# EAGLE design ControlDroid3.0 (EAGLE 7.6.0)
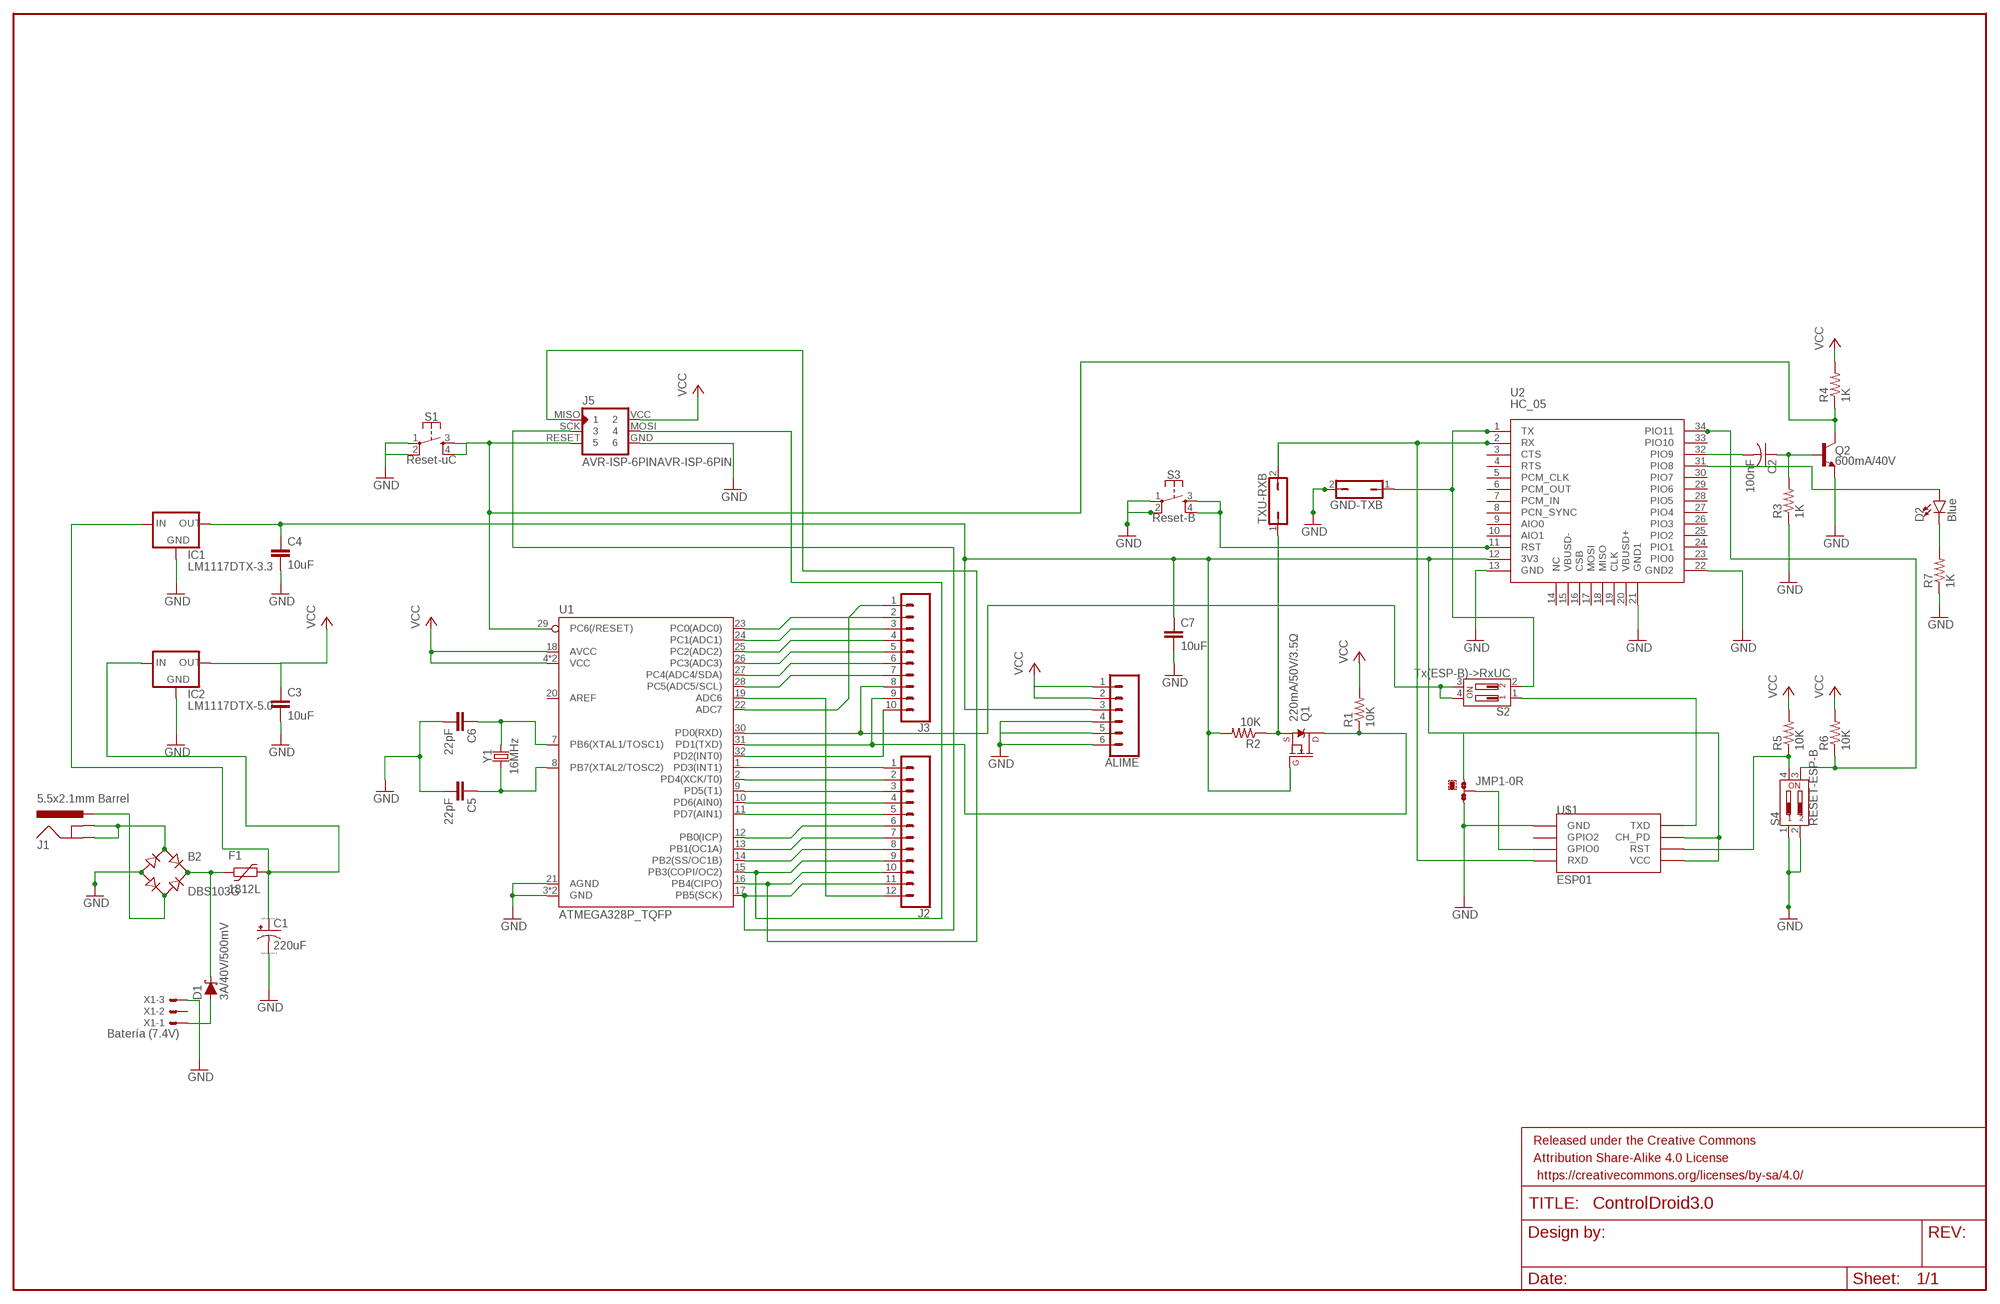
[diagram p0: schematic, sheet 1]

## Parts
ALIME  CONN_06NO_SILK_FEMALE_PTH  [1X06_NO_SILK]
B2  DBS103G  [DBS]
C1  220uF  CPOL-US153CLV-0605  [153CLV-0605]
C2  100nF  C-USC0805  [C0805]
C3  10uF  10UF-1206-6.3V-20%  [1206]
C4  10uF  10UF-1206-6.3V-20%  [1206]
C5  22pF  22PF-0603-50V-5%  [0603]
C6  22pF  22PF-0603-50V-5%  [0603]
C7  10uF  10UF-1206-6.3V-20%  [1206]
D1  3A/40V/500mV  DIODE-SCHOTTKY-B340A  [SMA-DIODE]
D2  Blue  LED-BLUE1206  [LED-1206]
F1  1812L  [1812L]
FRAME1  FRAME-LEDGERNO_FOOTPRINT  [DUMMY]
GND-TXB  JP1Q  [JP1]
IC1  LM1117DTX-3.3  [TO252]
IC2  LM1117DTX-5.0  [TO252]
J1  5.5x2.1mm Barrel  POWER_JACKSMD  [POWER_JACK_SMD]
J2  CONN_12  [1X12]
J3  CONN_10"  [1X10]
J5  AVR-ISP-6PINAVR-ISP-6PIN  [AVR-ISP-6PIN]
JMP1  0R-JUMPA  [A0R-JMP]
Q1  220mA/50V/3.5Ω  MOSFET-NCH-BSS138  [SOT23-3]
Q2  600mA/40V  TRANS_NPN-MMBT2222AL  [SOT23-3]
R1  10K  R-US_R1206  [R1206]
R2  10K  R-US_R1206  [R1206]
R3  1K  R-US_R1206  [R1206]
R4  1K  R-US_R1206  [R1206]
R5  10K  R-US_R1206  [R1206]
R6  10K  R-US_R1206  [R1206]
R7  1K  R-US_R1206  [R1206]
S1  Reset-uC  MOMENTARY-SWITCH-SPST-2-SMD-5.2MM  [TACTILE_SWITCH_SMD_5.2MM]
S2  Tx(ESP-B)->RxUC  DIP-02-SMD-50MIL-JWING  [DIPSWITCH-02-CHS-02A]
S3  Reset-B  MOMENTARY-SWITCH-SPST-2-SMD-5.2MM  [TACTILE_SWITCH_SMD_5.2MM]
S4  RESET-ESP-B  DIP-02-SMD-50MIL-JWING  [DIPSWITCH-02-CHS-02A]
TXU-RXB  JP1Q  [JP1]
U1  ATMEGA328P_TQFP  [TQFP32-08]
U2  HC_05  [BLUETOOTH_SMD]
U$1  ESP01  [ESP01]
X1  Batería (7.4V)  C-GRID-03-70543  [70543-03]
Y1  16MHz  CRYSTAL-8MHZSMD-HC49UP  [HC49UP]

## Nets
GND: ALIME.4 ALIME.5 ALIME.6 B2.- C1.- C3.2 C4.2 C5.2 C6.2 C7.2 GND-TXB.2 IC1.1(GND) IC2.1(GND) J5.GND JMP1.3 Q2.2(E) R3.1 R7.1 S1.1 S1.2 S3.1 S3.2 S4.1 S4.2 U1.3(GND) U1.5(GND) U1.21(AGND) U2.13(GND) U2.21(GND1) U2.22(GND2) U$1.GND X1.3
N$1: C6.1 U1.7(PB6(XTAL1/TOSC1)) Y1.2
N$2: B2.AC2 J1.VIN0(PWR)
N$3: B2.AC1 J1.GND(GNDBREAK) J1.P$4(GND)
N$4: B2.+ D1.C F1.P$1
N$6: C1.+ F1.P$2 IC1.2(IN) IC2.2(IN)
N$7: C5.1 U1.8(PB7(XTAL2/TOSC2)) Y1.1
N$8: J2.1 U1.1(PD3(INT1))
N$9: J2.2 U1.2(PD4(XCK/T0))
N$10: J2.3 U1.9(PD5(T1))
N$11: J2.4 U1.10(PD6(AIN0))
N$12: J2.5 U1.11(PD7(AIN1))
N$13: J2.6 U1.12(PB0(ICP))
N$14: J2.7 U1.13(PB1(OC1A))
N$15: J2.8 U1.14(PB2(SS/OC1B))
N$16: J2.9 J5.MOSI U1.15(PB3(COPI/OC2))
N$17: J3.9 Q1.3(D) R1.1 U1.31(PD1(TXD))
N$18: J2.11 J5.SCK U1.17(PB5(SCK))
N$19: J2.12 U1.19(ADC6)
N$20: J3.1 U1.22(ADC7)
N$21: J3.2 U1.23(PC0(ADC0))
N$22: J3.3 U1.24(PC1(ADC1))
N$23: J3.4 U1.25(PC2(ADC2))
N$24: J3.5 U1.26(PC3(ADC3))
N$25: J3.6 U1.27(PC4(ADC4/SDA))
N$26: J3.7 U1.28(PC5(ADC5/SCL))
N$27: S2.1 U$1.TX(TXD)
N$28: J3.8 S2.3 S2.4 U1.30(PD0(RXD))
N$29: J3.10 U1.32(PD2(INT0))
N$30: Q1.2(S) R2.1 TXU-RXB.1
N$32: J5.RESET Q2.3(C) R4.1 S1.3 S1.4 U1.29(PC6(/RESET))
N$35: D1.A X1.1
N$36: ALIME.3 C4.1 C7.1 IC1.TAB(OUT) JMP1.1 Q1.1(G) R2.2 U2.12(3V3) U$1.CH_PD U$1.VCC
N$37: J2.10 J5.MISO U1.16(PB4(CIPO))
N$38: GND-TXB.1 S2.2 U2.1(TX)
N$39: TXU-RXB.2 U2.2(RX) U$1.RX(RXD)
N$40: S3.3 S3.4 U2.11(RST)
N$41: C2.2 U2.32(PIO9)
N$42: C2.1 Q2.1(B) R3.2
N$43: R5.1 S4.4 U$1.RST
N$44: R6.1 S4.3 U2.34(PIO11)
N$45: D2.A U2.31(PIO8)
N$46: D2.C R7.2
N$47: JMP1.2 U$1.GPIO0
VCC: ALIME.1 ALIME.2 C3.1 IC2.TAB(OUT) J5.VCC R1.2 R4.2 R5.2 R6.2 U1.4(VCC) U1.6(VCC) U1.18(AVCC)
Unconnected: U1.20(AREF) U2.3(CTS) U2.4(RTS) U2.5(PCM_CLK) U2.6(PCM_OUT) U2.7(PCM_IN) U2.8(PCN_SYNC) U2.9(AIO0) U2.10(AIO1) U2.14(NC) U2.15(VBUSD-) U2.16(CSB) U2.17(MOSI) U2.18(MISO) U2.19(CLK) U2.20(VBUSD+) U2.23(PIO0) U2.24(PIO1) U2.25(PIO2) U2.26(PIO3) U2.27(PIO4) U2.28(PIO5) U2.29(PIO6) U2.30(PIO7) U2.33(PIO10) U$1.GPIO2 X1.2

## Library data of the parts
ALIME = SparkFun-Connectors:CONN_06: Multi connection point. Often used as Generic Header-pin footprint for 0.1 inch spaced/style header connections On any of the 0.1 inch spaced packages, you can populate with these: Break Away Headers - Straight (PRT-00116) Break Away Male Headers - Right Angle (PRT-00553) Female Headers (PRT-00115)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; PROD_ID: CONN-08437
B2 = rectifier:DB?*G: Single Phase 1.0 AMP Glass Passivated Bridge Rectifier Taiwan Semiconductor Co.,Ltd. - TSC Source: http://www.taiwansemi.com/TSCbig5/ezcatfiles/cust/img/img/db101g.pdf http://www.ts.com.tw/db/pictures/modules/PDT/PDT060207001/DBLS201G.pdf
C1 = resistor:CPOL-US: POLARIZED CAPACITOR, American symbol
C2 = rcl:C-US: CAPACITOR, American symbol
C3 C4 C7 = SparkFun-Capacitors:10UF: 10.0µF ceramic capacitors; PROD_ID: CAP-10057
C5 C6 = SparkFun-Capacitors:22PF: 22pF ceramic capacitors; PROD_ID: CAP-07876
D1 = SparkFun-DiscreteSemi:DIODE-SCHOTTKY: Schottky diode; PROD_ID: DIO-09886
D2 = SparkFun-LED:LED-BLUE: Blue SMD LED; PROD_ID: DIO-09911
F1 = ptc-littlefuse:1812L
FRAME1 = SparkFun-Aesthetics:FRAME-LEDGER: Schematic Frame - Ledger
GND-TXB TXU-RXB = jumper:JP1Q: JUMPER
IC1 IC2 = lm1117:LM1117DTX-*
J1 = SparkFun-Connectors:POWER_JACK: Power Jack Connector This is the standard 5.5mm barrel jack for power. The PTH is the most common, proven, reliable, footprint. The Slot footprint only works if the mill layer is transmitted to the PCB fab house so be warned. Here are the connectors we sell at SparkFun: DC Barrel Power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; PROD_ID: CONN-08106; SF_ID: PRT-12748
J2 = SparkFun-Connectors:CONN_12: Multi connection point. Often used as Generic Header-pin footprint for 0.1 inch spaced/style header connections On any of the 0.1 inch spaced packages, you can populate with these: Break Away Headers - Straight (PRT-00116) Break Away Male Headers - Right Angle (PRT-00553) Female Headers (PRT-00115)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
J3 = SparkFun-Connectors:CONN_10: Multi connection point. Often used as Generic Header-pin footprint for 0.1 inch spaced/style header connections On any of the 0.1 inch spaced packages, you can populate with these: Break Away Headers - Straight (PRT-00116) Break Away Male Headers - Right Angle (PRT-00553) Female Headers (PRT-00115)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; PROD_ID: CONN-11563
J5 = avr-isp:AVR-ISP-6PIN: AVR ISP 6pin 3x2 pin header
JMP1 = jump-0r-smd:0R-JUMP: SMD 0R 0805 Jumper
Q1 = SparkFun-DiscreteSemi:MOSFET-NCH: N-channel MOSFETs Voltage controlled devices that allow control of high current outputs. SparkFun Products: SparkFun OpenScale SparkFun Digital Sandbox SparkFun Monster Moto Shield SparkFun MOSFET Power Controller; PROD_ID: TRANS-00830
Q2 = SparkFun-DiscreteSemi:TRANS_NPN: NPN transistor Current controlled devices typically used to amplify current or used as a switch. BC547 - COM-08928 (TO-92 45V 100mA) (1.Collector 2.Base 3.Emitter) 2N3904 - COM-00521 (TO-92 40V 200mA) (1.Emitter 2.Base 3.Collector) P2N2222A - COM-12852 (TO-92 40V 600mA) (1.Collector 2.Base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; PROD_ID: TRANS-08049
R1-R7 = resistor:R-US_: RESISTOR, American symbol
S1 S3 = SparkFun-Switches:MOMENTARY-SWITCH-SPST-2: Momentary Switch (Pushbutton) - SPST - Two Circuits Normally-open (NO) SPST momentary switches (buttons, pushbuttons). Schematic symbol includes two switch circuits. Variants SMD-4.6MMX2.8MM - 4.60mm x 2.80mm Tactile Momentary Button Switch - Used on SparkFun Pro Micro - RP2040 SMD-5.2MM - Mini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; PROD_ID: SWCH-08247; SF_SKU: COM-08720
S2 S4 = SparkFun-Switches:DIP-02: 2-Position DIP Switch 2-circuit DIP (dual inline package) switch. Commonly used to physcially set a circuit's behavior. Variants PTH-100MIL - Through-hole, 0.1"-Pitch Used on SparkFun Stepoko (ROB-13899) SMD-50MIL-JWING - SMD (J-Wing Pads), 0.05"-Pitch Prototype Part SMD-50MIL - SMD, 0.05"-Pitch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; PROD_ID: SWCH-12372
U1 = SparkFun-IC-Microcontroller:ATMEGA328P_TQFP: Popular 328P in QFP Storefront component: ATmega328 - TQFP (COM-13448) Datasheet SparkFun Products SparkFun RedBoard - Programmed with Arduino (DEV-12757) Arduino Pro Mini 328 - 5V/16MHz (DEV-11113) Arduino Pro Mini 328 - 3.3V/8MHz (DEV-11114) SparkFun OpenLog (DEV-13712) SparkFun MicroView - OLED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; PROD_ID: IC-09069
U2 = Bluetooth HC-05:HC_05: HC-05 Bluetooth Module
U$1 = esp8266modules:ESP01: ESP8266 Wifi module 01
X1 = con-molex:C-GRID-03: CONNECTOR wire to board 2.54 mm (0.100") pitch header; OC_FARNELL: unknown; OC_NEWARK: unknown
Y1 = SparkFun-Clocks:CRYSTAL-8MHZ: 8MHz Crystal; PROD_ID: XTAL-11706; VALUE: 8MHz

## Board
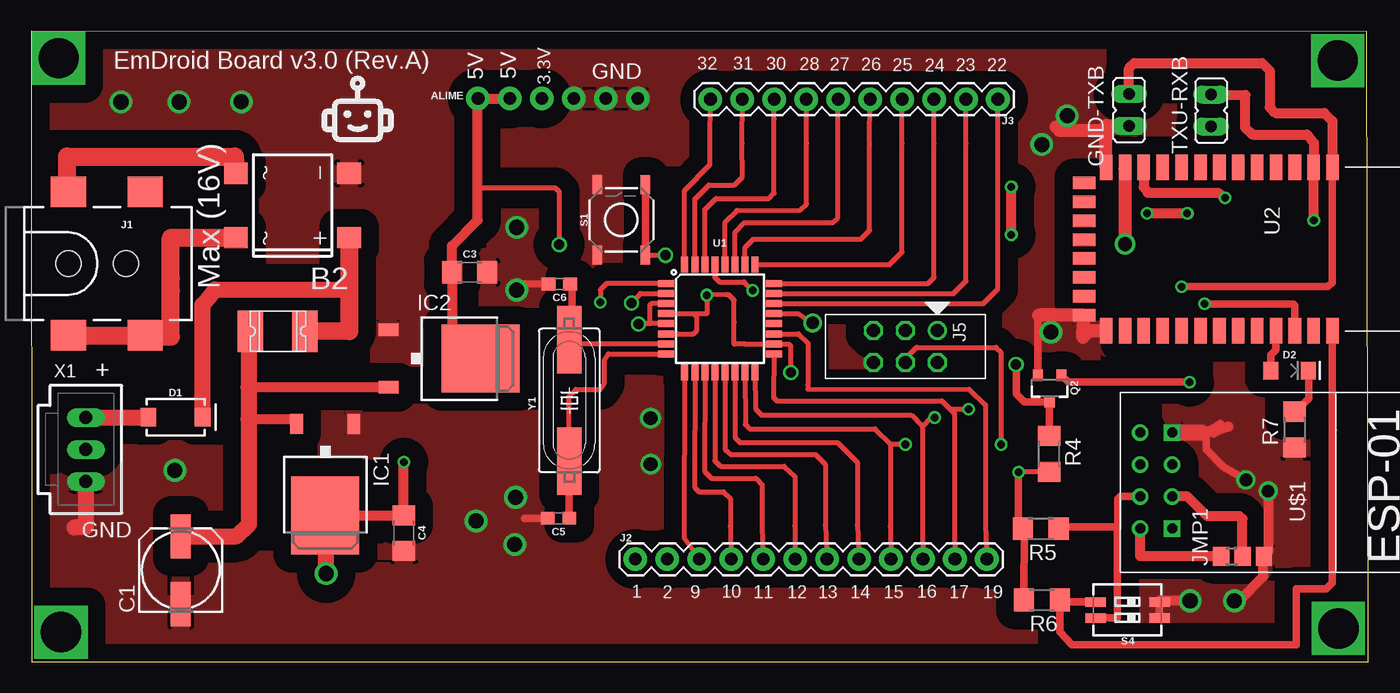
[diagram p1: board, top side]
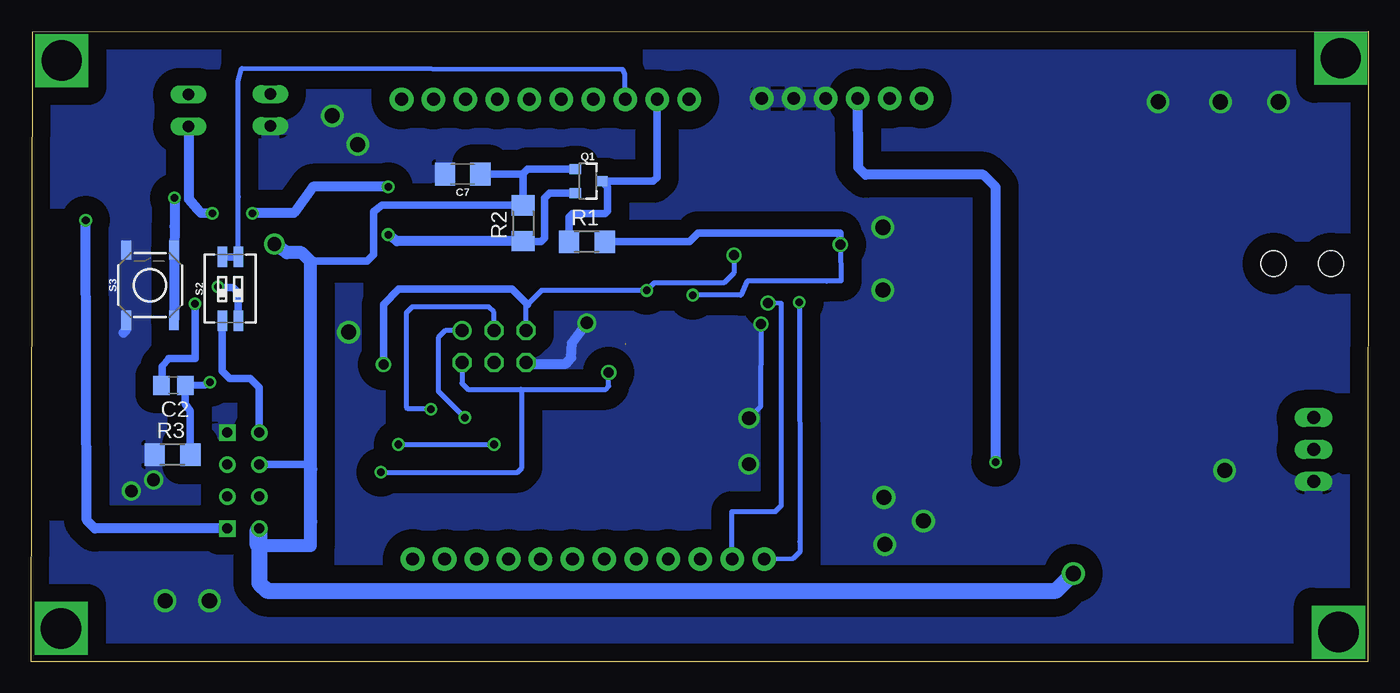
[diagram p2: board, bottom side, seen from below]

Size 106.24 x 50.1 mm. Coordinates in mm from the lower left corner, seen from the top.
Outline: 0,0 106.24,0 106.15,50.06 0,50.1 0,0
Copper layers (1*16): Top 0.035mm / dielectric 1.5mm / Bottom 0.035mm
Design rules "default *": minimum track width 10mil, minimum drill 16mil, track to track 8mil, track to pad 8mil, pad to pad 8mil, via to via 8mil, smd to smd 8mil, copper to edge 40mil, drill to drill 8mil, minimum pad ring 10mil, minimum via ring 8mil, stop-mask expansion 4mil, vias tented up to drill 0mil, thermal gap 10mil

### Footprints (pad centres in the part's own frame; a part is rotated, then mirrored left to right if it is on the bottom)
1X06_NO_SILK = drill 1.016 pad 1.88: 1 0,0; 2 2.54,0; 3 5.08,0; 4 7.62,0; 5 10.16,0; 6 12.7,0
DBS = smd 1.7 x 1.9: + -2.55,-4.5; - 2.55,-4.5; AC1 -2.55,4.5; AC2 2.55,4.5
153CLV-0605 = smd 3.5 x 1.6: + 2.7,0; - -2.7,0
C0805 = smd 1.3 x 1.5: 1 -0.95,0; 2 0.95,0
1206 = smd 1.6 x 1.8: 1 -1.4,0; 2 1.4,0
0603 = smd 1.1 x 1: 1 -0.85,0; 2 0.85,0
SMA-DIODE = smd 1.27 x 1.47: A -2.15,0; C 2.15,0
LED-1206 = smd 1.2 x 1.4: A -1.5,0; C 1.5,0
1812L = smd 2.03 x 3.3: P$1 -2.16,0; P$2 2.16,0
JP1 = drill 0.914 long: 1 0,-1.27; 2 0,1.27
TO252 = smd 1 x 1.6: 1 -2.28,-4.8; 2 2.28,-4.8 | smd 5.4 x 6.2: TAB 0,2.5
POWER_JACK_SMD = smd 2.8 x 2.4: GND 0,-5.7; P$4 6.1,-5.7; VIN0 0,5.7; VIN1 6.1,5.7 | hole 2.032: 0,0; 4.572,0
1X12 = drill 1.016 pad 1.88: 1 0,0; 2 2.54,0; 3 5.08,0; 4 7.62,0; 5 10.16,0; 6 12.7,0; 7 15.24,0; 8 17.78,0; 9 20.32,0; 10 22.86,0; 11 25.4,0; 12 27.94,0
1X10 = drill 1.016 pad 1.88: 1 0,0; 2 2.54,0; 3 5.08,0; 4 7.62,0; 5 10.16,0; 6 12.7,0; 7 15.24,0; 8 17.78,0; 9 20.32,0; 10 22.86,0
AVR-ISP-6PIN = drill 1.016 octagon: GND 1.27,-2.54; MOSI 1.27,0; RESET -1.27,-2.54; SCK -1.27,0; VCC 1.27,2.54 | drill 1.016: MISO -1.27,2.54
A0R-JMP = smd 1.5 x 1.3: 1 0,1.7; 2 0,0; 3 0,-1.7
SOT23-3 = smd 0.8 x 0.9: 1 -0.95,-1; 2 0.95,-1; 3 0,1.1
R1206 = smd 1.6 x 1.803: 1 -1.422,0; 2 1.422,0
TACTILE_SWITCH_SMD_5.2MM = smd 1.524 x 0.762: 1 -2.794,1.905; 2 2.794,1.905; 3 -2.794,-1.905; 4 2.794,-1.905
DIPSWITCH-02-CHS-02A = smd 0.76 x 1.6: 1 0,-2.54; 2 1.27,-2.54; 3 1.27,2.54; 4 0,2.54
TQFP32-08 = smd 1.27 x 0.559: 1 -4.293,2.8; 2 -4.293,2; 3 -4.293,1.2; 4 -4.293,0.4; 5 -4.293,-0.4; 6 -4.293,-1.2; 7 -4.293,-2; 8 -4.293,-2.8; 17 4.293,-2.8; 18 4.293,-2; 19 4.293,-1.2; 20 4.293,-0.4; 21 4.293,0.4; 22 4.293,1.2; 23 4.293,2; 24 4.293,2.8 | smd 0.559 x 1.27: 9 -2.8,-4.293; 10 -2,-4.293; 11 -1.2,-4.293; 12 -0.4,-4.293; 13 0.4,-4.293; 14 1.2,-4.293; 15 2,-4.293; 16 2.8,-4.293; 25 2.8,4.293; 26 2,4.293; 27 1.2,4.293; 28 0.4,4.293; 29 -0.4,4.293; 30 -1.2,4.293; 31 -2,4.293; 32 -2.8,4.293
BLUETOOTH_SMD = smd 2 x 1: 1 -6.35,3.81; 2 -6.35,2.31; 3 -6.35,0.81; 4 -6.35,-0.69; 5 -6.35,-2.19; 6 -6.35,-3.69; 7 -6.35,-5.19; 8 -6.35,-6.69; 9 -6.35,-8.19; 10 -6.35,-9.69; 11 -6.35,-11.19; 12 -6.35,-12.69; 13 -6.35,-14.19; 22 6.65,-14.19; 23 6.65,-12.69; 24 6.65,-11.19; 25 6.65,-9.69; 26 6.65,-8.19; 27 6.65,-6.69; 28 6.65,-5.19; 29 6.65,-3.69; 30 6.65,-2.19; 31 6.65,-0.69; 32 6.65,0.81; 33 6.65,2.31; 34 6.65,3.81 | smd 1 x 1.8: 14 -5.1,-15.94; 15 -3.6,-15.94; 16 -2.1,-15.94; 17 -0.6,-15.94; 18 0.9,-15.94; 19 2.4,-15.94; 20 3.9,-15.94; 21 5.4,-15.94
ESP01 = drill 0.8: CH_PD -1.285,-8.178; GPIO0 1.255,-5.638; GPIO2 -1.285,-5.638; RST 1.255,-8.178; TX -3.825,-8.178; VCC 3.795,-8.178 | drill 0.8 square: GND -3.825,-5.638; RX 3.795,-5.638
70543-03 = drill 1.016 long: 1 -2.54,0; 2 0,0; 3 2.54,0
HC49UP = smd 5.334 x 1.93: 1 -4.826,0; 2 4.826,0

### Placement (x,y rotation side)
ALIME  35.49,44.77 0 top
B2  20.75,36.26 90 top
C1  11.87,7.27 90 top
C2  94.97,21.96 180 bottom
C3  34.83,30.95 0 top
C4  29.59,10.21 270 top
C5  41.9,11.39 180 top
C6  41.96,30.02 180 top
C7  71.97,38.76 180 bottom
D1  11.45,19.42 0 top
D2  100,23.14 0 top
F1  19.58,26.26 180 top
FRAME1  -2.16,-0.19 0 top
GND-TXB  87.25,43.86 180 top
IC1  23.36,14.11 180 top
IC2  33.18,24.09 270 top
J1  2.94,31.64 0 top
J2  48,8.14 0 top
J3  76.82,44.71 180 top
J5  69.47,25.05 270 top
JMP1  96.25,8.37 90 top
Q1  62.02,38.2 270 bottom
Q2  80.93,21.76 180 top
R1  62.09,33.39 0 bottom
R2  67.16,34.85 90 bottom
R3  95.03,16.46 0 bottom
R4  80.9,16.51 270 top
R5  80.23,10.57 180 top
R6  80.32,4.91 180 top
R7  100.39,18.44 90 top
S1  46.9,35.12 90 top
S2  91.08,29.64 0 bottom
S3  96.81,29.93 90 bottom
S4  87.13,3.46 90 top
TXU-RXB  93.76,43.82 0 top
U1  54.73,27.26 0 top
U2  99.61,32.95 270 top
U$1  96.31,14.38 270 top
X1  4.32,16.86 270 top
Y1  42.75,20.76 90 top

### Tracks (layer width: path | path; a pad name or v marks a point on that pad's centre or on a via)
GND  (via drill 0.8, 1, 1.1, 1.2)
  Top 0.406: v62.1,26.92 60.93,27.66 U1.21 | U1.5 49.16,26.86 | 49.16,26.86 48.87,26.86 v48.25,26.85 | U1.3 49.28,28.46 49.14,28.32 49.14,26.89 49.16,26.86
  Top 0.61: C6.2 38.32,30.06 | C5.2 39.19,11.37 | Q2.2 79.98,27.45 80.06,27.52 | S4.1 S4.2 | v96.54,14.44 94.71,15.52 93.37,16.86 93.37,18.29 | 94.5,18.93 93.37,18.29 | 93.37,18.29 95.15,18.67
  Top 0.813: GND-TXB.2 85.41,42.72 84.91,42.23 | 93.01,18.2 95.15,18.67 93.96,18.2 94.08,18.32 | 93.02,18.2 94.55,18.55 | v92.09,4.83 89.67,4.83 S4.2 | v98.3,13.56 98.3,8.72 JMP1.3 97.93,8.35 97.93,6.77 96,4.83 v95.62,4.83
  Top 1.016: U2.21 83.54,25.85 83.59,25.8 84.09,26.3 U2.22 | U2.21 83.54,26.03 83.59,25.98 | 85.36,42.14 85.42,42.61 U2.13 85.42,42.26 85.13,42.23 84.91,42.23 81.73,42.23 81.46,42.5 | U2.21 80.08,27.55 80.06,27.52
  Top 1.27: X1.3 4.32,10.67 3.43,10.66 | U$1.GND 93.01,18.2 93.02,18.2
  Bottom 0.406: v62.1,26.92 61.64,26.82 61.74,26.72 | v48.25,26.85 48.28,20.29 v49.22,19.35
  Bottom 0.813: 66.89,23.62 66.93,23.42 J5.GND 67.03,23.47 66.96,23.66 63.76,23.66 63.34,24.14 63.28,25.31 v62.1,26.92 | S3.1 98.71,26.37 98.93,26.15
  other vias: 16.68,44.51 38.57,34.53 49.22,15.69 38.42,9.3 38.57,29.54 7.11,44.5 38.48,13.05 80.31,41.12 82.34,43.4 35.35,11.17 11.73,44.5 81.03,26.19 11.4,15.2
  pour Top (isolate 1.422): 0.14,49.78 107.14,49.78 107.98,0.63 0.98,0.63
  pour Bottom (isolate 1.422): 0.45,49.69 107.95,49.69 107.82,0.52 0.32,0.52
N$1
  Top 0.406: U1.7 42.75,25.26 Y1.2
  Top 0.61: Y1.2 42.95,27.76 42.95,30.02 C6.1
N$2
  Top 1.422: J1.VIN0 2.85,37.86 2.83,40.15 16.17,40.17 B2.AC2
N$3
  Top 1.422: J1.GND J1.P$4 | J1.P$4 9.44,25.75 9.04,25.92 8.8,25.95 J1.P$4 | J1.P$4 9.12,25.79 9.28,25.89 9.12,25.84 11.07,25.83 11.08,29.46 11.07,30.48 11.07,33.71 B2.AC1
N$4
  Top 1.27: D1.C 13.6,28.35 14.6,29.58 24.89,29.58 25.25,28.98
  Top 1.422: B2.+ 25.25,28.98 25.25,27.63 25.26,26.26 F1.P$1
N$5  (via drill 3.2)
  other vias: 2.35,2.34
N$6
  Top 0.813: 17.26,19.27 20.71,19.27 IC1.2 | IC2.2 17.26,21.81 | F1.P$2 17.26,26.26
  Top 1.27: 17.26,26.26 17.26,21.81 17.26,19.27 17.3,19.23 17.29,10.9 16.31,9.97 C1.+
N$7
  Top 0.406: Y1.1 42.73,20.25 42.73,21.1 43.28,21.64 45.21,21.64 45.25,21.68 45.55,22.13 45.55,23.97 45.86,24.46 50.46,24.46 U1.8
  Top 0.61: Y1.1 C5.1
N$8  (via drill 0.6)
  Top 0.406: U1.1 45.72,30.06 45.23,29.56 v45.21,28.56
  Bottom 0.406: v45.21,28.56 45.17,9.55 45.17,8.72 45.72,8.17 J2.1
N$9  (via drill 0.8)
  Top 0.406: v47.7,28.51 47.75,28.62 48.41,29.26 50.46,29.26 U1.2
  Bottom 0.406: J2.2 50.56,11.94 47.09,11.94 46.63,12.42 46.63,28.48 v47.7,28.51
N$10
  Top 0.406: U1.9 51.89,9.84 J2.3
N$11
  Top 0.406: U1.10 52.72,13.85 53.06,13.5 55.02,13.5 55.56,12.97 55.56,10.78 J2.4
N$12
  Top 0.406: U1.11 53.51,15.13 54.04,14.57 57.58,14.57 58.08,14.06 58.08,10.79 J2.5
N$13
  Top 0.406: U1.12 54.32,15.96 54.77,15.52 59.83,15.52 60.69,14.74 60.69,10.8 J2.6
N$14
  Top 0.406: U1.13 55.14,16.88 55.59,16.45 62.32,16.45 63.11,15.66 63.11,10.84 J2.7
N$15
  Top 0.406: U1.14 55.92,17.82 56.32,17.42 64.06,17.42 65.65,15.83 65.65,10.85 J2.8
N$16  (via drill 0.6)
  Top 0.406: U1.15 56.75,18.83 57.08,18.51 67.06,18.51 68.28,17.3 | 68.28,17.3 68.28,10.76 J2.9 | J5.MOSI 69.47,24.09 70.36,24.98 76.68,24.98 77.05,24.61 77.05,17.29 v77.07,17.26 | v69.47,17.26 68.31,17.26 68.28,17.3
  Bottom 0.406: v77.07,17.26 v69.47,17.26
N$17
  Top 0.406: U1.31 52.73,36.78 53.85,37.9 55.87,37.9 56.52,38.53 56.5,41.18 J3.9
  Bottom 0.61: J3.9 56.52,42.54 56.51,38.48 56.82,38.2 Q1.3 60.45,37.73 60.45,35.82 60.65,35.63 63.23,35.63 63.52,35.34 R1.1
N$18  (via drill 0.6)
  Top 0.406: U1.17 58.99,20.98 59.25,20.74 72.36,20.74 73.14,19.95 | 73.14,19.95 73.37,19.72 73.37,10.78 J2.11 | v74.49,20.06 73.24,20.06 73.14,19.95
  Bottom 0.406: J5.SCK 69.47,27.78 69.89,28.2 75.98,28.2 76.46,27.72 76.46,20.22 76.38,20.14 74.57,20.14 v74.49,20.06
N$19
  Top 0.406: U1.19 60.98,26.06 61.73,25.32 61.72,21.97 61.71,21.65 74.55,21.64 75.84,20.41 75.84,10.82 J2.12
N$20
  Top 0.406: U1.22 75.67,28.46 76.8,29.6 76.8,41.19 J3.1
N$21
  Top 0.406: U1.23 73.3,29.26 74.28,30.24 74.28,41.21 J3.2
N$22
  Top 0.406: U1.24 71.26,30.06 71.74,30.54 71.74,41.2 J3.3
N$23
  Top 0.406: U1.25 68.2,31.55 69.19,32.54 69.19,41.2 J3.4
N$24
  Top 0.406: U1.26 56.72,32.93 57.39,33.57 65.92,33.57 66.62,34.28 66.62,41.17 J3.5
N$25
  Top 0.406: U1.27 55.92,34.13 56.66,34.89 63.67,34.89 64.09,35.27 64.09,41.02 J3.6
N$26
  Top 0.406: U1.28 55.13,34.94 56.07,35.86 61.07,35.89 61.61,36.39 61.61,41.22 J3.7
N$27
  Bottom 0.61: 88.11,18.25 88.1,18.22 U$1.TX 88.13,21.78 88.87,22.52 90.51,22.52 91.08,23.09 S2.1
N$28
  Top 0.406: U1.30 53.53,35.94 54.41,36.82 58.6,36.82 59.02,37.24 59.02,43.15 J3.8
  Bottom 0.406: S2.3 89.81,36.96 89.82,36.98 89.82,46.13 89.52,47.17 59.26,47.1 59.09,46.71 59.09,44.67 J3.8
  Bottom 0.61: S2.4 S2.3
N$29
  Top 0.406: U1.32 51.93,37.45 53.92,39.5 53.92,41.26 J3.10
N$30  (via drill 0.6)
  Top 0.813: v77.89,33.95 v77.89,37.75 | v88.68,35.65 91.72,35.65 v91.87,35.63
  Bottom 0.61: Q1.2 65.06,37.25 65.46,36.85 65.46,33.68 65.74,33.4 67.13,33.4 R2.1
  Bottom 0.813: R2.1 77.18,33.43 v77.89,33.95 | v77.89,37.75 83.87,37.75 85.37,35.67 v88.68,35.65 | TXU-RXB.1 93.73,36.76 93.06,35.98 92.77,35.66 v91.87,35.63
N$31  (via drill 3.2)
  other vias: 2.16,47.97
N$32  (via drill 0.6, 0.8)
  Top 0.406: U1.29 54.33,30.54 54.67,30.19 56.65,30.19 v57.34,29.5 | S1.3 50.39,32.33 v50.41,32.3
  Top 0.61: S1.4 S1.3 | v78.26,23.62 78.3,23.59 78.3,21.3 78.94,20.66 Q2.3 80.9,20.62 R4.1
  Bottom 0.406: J5.RESET 66.96,26.34 66.96,28.24 66.82,28.38 65.7,29.5 v57.34,29.5 56.75,30.1 51.21,30.1 50.41,30.91 v50.41,32.3
  Bottom 0.61: v78.26,23.62 78.26,28.39 77.04,29.61 68.05,29.61 66.82,28.38
N$33  (via drill 3.2)
  other vias: 103.84,47.79
N$34  (via drill 3.2)
  other vias: 103.89,2.63
N$35
  Top 1.27: X1.1 9.28,19.4 D1.A
N$36  (via drill 0.6, 1.1, 1.2)
  Top 0.813: IC1.TAB C4.1 v29.59,15.85 v29.6,15.85 | JMP1.1 88.13,8.37 U$1.VCC
  Top 1.016: v86.93,33.19 86.93,39.13 U2.12
  Top 1.27: v23.42,7 23.42,11.54 IC1.TAB
  Bottom 0.61: Q1.1 66.83,39.15 67.18,38.8 | 67.18,38.8 67.18,36.29 | 67.18,36.29 R2.2 | 67.18,36.29 78.37,36.29 79.04,35.77 79.04,32.36 79.56,31.83 84.01,31.83 84.04,31.79 | C7.1 67.22,38.76 67.18,38.8 | U$1.CH_PD 84.4,15.66 84.04,15.3
  Bottom 0.813: v29.6,15.85 29.6,37.71 30.59,38.7 39.94,38.7 40.51,39.28 40.51,41.25 ALIME.3
  Bottom 1.016: 88.25,9.24 84.06,9.22 84.04,11.14 84.04,15.3 84.04,31.79 84.77,32.52 85.95,32.52 v86.93,33.19
  Bottom 1.27: v23.42,7 24.8,5.62 87.52,5.62 88.13,6.24 U$1.VCC 88.25,10.46 88.25,9.24
N$37  (via drill 0.6)
  Top 0.406: U1.16 57.55,20.1 58.05,19.6 69.93,19.6 70.82,18.71 | 70.82,18.71 70.82,10.77 J2.10 | v71.8,19.4 71.51,19.4 70.82,18.71
  Bottom 0.406: J5.MISO 73.36,26.31 73.91,25.76 73.91,21.51 v71.8,19.4
N$38  (via drill 0.6)
  Top 0.61: v91.42,29.8 103.03,29.8 103.38,30.14 103.38,39.2 U2.1
  Top 0.813: GND-TXB.1 87.25,47.18 87.67,47.59 97.83,47.59 98.43,46.99 98.43,44.07 98.87,43.62 102.78,43.62 103.41,42.99 U2.1
  Bottom 0.61: S2.2 89.81,29.33 90.2,29.73 91.34,29.73 v91.42,29.8
N$39  (via drill 0.6)
  Top 0.813: TXU-RXB.2 96.49,45.04 96.46,45.04 96.46,42.46 97.03,41.9 101.41,41.9 101.93,41.23 101.94,39.9 | 101.94,39.9 101.94,39.31 U2.2 | v101.93,35.08 101.93,39.94 101.94,39.9
  Bottom 0.813: U$1.RX 101.2,10.58 101.84,11.23 v101.93,35.08
N$40  (via drill 0.6)
  Top 0.813: U2.11 88.42,37.72 88.72,37.29 94.34,37.29 v94.87,36.88
  Bottom 0.813: v94.87,36.88 94.87,34.62 S3.4 S3.3
N$41  (via drill 0.6)
  Top 0.61: U2.32 100.42,28.32 100.29,28.44 v93.25,28.44
  Bottom 0.61: v93.25,28.44 93.23,24.09 95.35,24.08 95.85,23.44 95.85,21.9 95.86,21.75 C2.2
N$42  (via drill 0.6)
  Top 0.61: v92.06,22.21 82.43,22.21 Q2.1
  Bottom 0.61: v92.06,22.21 92.07,22.26 92.49,21.98 C2.1 94.03,20.49 93.62,19.91 R3.2
N$43
  Top 0.61: S4.4 86.33,3.47 86.32,4.55 86.32,10.72 | 86.32,10.72 82.14,10.71 R5.1 | U$1.RST 86.54,13.12 86.35,12.94 86.35,10.59 86.32,10.72
N$44
  Top 0.61: S4.3 81.87,4.73 81.86,5.12 81.61,5.21 R6.1 81.76,3.96 81.76,2.37 82.69,1.33 99.06,1.33 100.53,1.33 100.53,5.8 102.94,5.78 103.42,6.25 103.42,7.6 103.42,18.46 | U2.34 103.42,18.46 | 103.42,18.46 103.47,18.4
N$45
  Top 0.61: D2.A 98.5,24.37 98.91,24.78 98.91,26.29 U2.31
N$46
  Top 0.61: R7.2 100.45,19.87 101.52,20.94 101.52,23.12 D2.C
N$47
  Top 0.813: JMP1.2 96.25,11.35 96.05,11.55 93.47,11.55 91.89,13.13 U$1.GPIO0
VCC  (via drill 0.6, 0.8)  (1 unrouted)
  Top 0.254: 55.85,26.75 55.86,26.99
  Top 0.406: v41.95,33.16 41.95,37.36 41.65,37.66 35.49,37.66 35.46,37.63 | 50.54,27.65 52.92,27.65 53.68,27.65 v53.69,29.14 55.25,29.17 55.43,29.15 55.86,28.74 55.86,26.99 55.86,25.25 56.74,25.25 59,25.25 U1.18 | v60.36,22.98 60.36,25.11 60.24,25.23 59.05,25.23 | R4.2 78.5,15.09 v78.46,15.05 | 50.54,27.65 52.63,27.65 52.86,27.42 52.86,26.3 52.58,26.01 50.48,26.01 U1.6 | 50.54,27.65 U1.4
  Top 0.61: R6.2 78.94,10.71 R5.2 78.46,10.92 v78.46,15.05
  Top 0.813: IC2.TAB 33.43,26.34 C3.1 33.43,33.05 35.46,35.08 35.46,37.63 35.46,44.74 ALIME.1 ALIME.2
  Bottom 0.406: v41.95,33.16 41.88,30.26 43.01,30.25 49.35,30.24 49.86,29.14 v53.69,29.14 | J5.VCC 72.01,22.11 71.54,21.64 67.34,21.64 | 67.34,21.64 60.59,21.64 60.36,21.88 v60.36,22.98 | v78.46,15.05 67.6,15.05 67.25,15.4 67.25,21.54 67.34,21.64
  Bottom 0.61: R1.2 53.93,33.38 53.25,34.06 41.98,34.08 v41.95,33.16

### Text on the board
tPlace: EmDroid Board v3.0 (Rev.A)
tNames: 32 | 31 | 30 | 28 | 27 | 26 | 25 | 24 | 23 | 22 | 5V | 5V | 3.3V | GND | Max (16V) | + | GND | 1 | 2 | 9 | 10 | 11 | 12 | 13 | 14 | 15 | 16 | 17 | 19

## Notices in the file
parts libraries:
SparkFun-Connectors: Licensing: Creative Commons ShareAlike 4.0 International - https://creativecommons.org/licenses/by-sa/4.0
SparkFun-Aesthetics: Released under the Creative Commons Attribution Share-Alike 4.0 License
SparkFun-Aesthetics: https://creativecommons.org/licenses/by-sa/4.0
